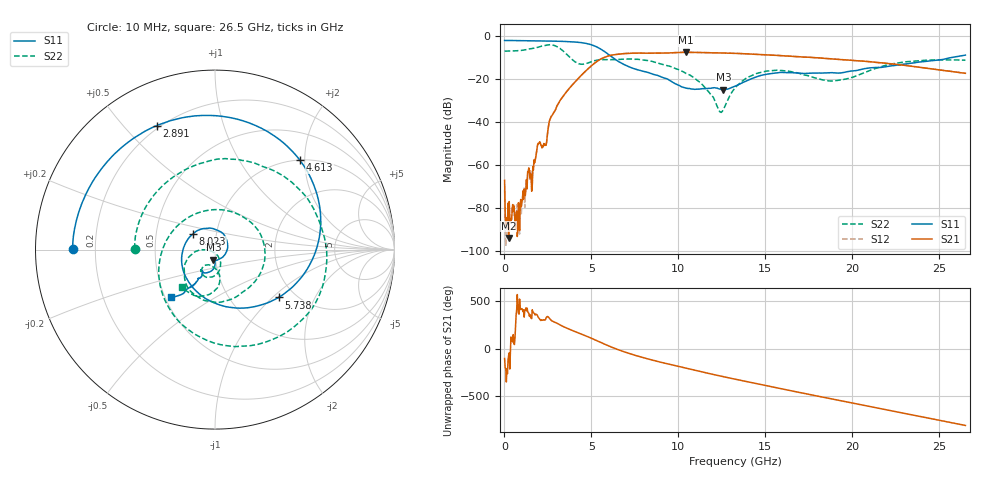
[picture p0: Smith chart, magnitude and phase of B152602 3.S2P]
!  2-Port S-parameters saved by WinCal
! VAR MeasName=S-Parameters (CALIBRATED_DATA) read from VNA (N5242A)
! VAR MeasDate=2016-1-5 16:25:45
! VAR NAME=B152602 3
! VAR FILENAME=B152602 3.S2P
! VAR DATE=2016-1-5 16:25:45
! VAR PHYS_PORTS=1,2
# Hz S DB R 50
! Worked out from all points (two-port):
!   801 points, 10 MHz to 26.5 GHz, reference 50 ohm
!   highest |S21| = -7.52 dB at 10.44 GHz (marker M1); lowest = -93.8 dB at 241.8 MHz (marker M2)
!   |S21| within 3 dB of the highest: 5.573 GHz to 18.72 GHz (13.14 GHz wide, 108 % of centre)
!   lowest |S11| = -24.9 dB at 12.59 GHz (marker M3), VSWR 1.12, Z = 48.8 - j5.54 ohm
!   |S11| at or under -10 dB: 6.233 GHz to 25.66 GHz (19.43 GHz wide, 122 % of centre)
!   |S22| runs from -35.5 to -4.0 dB; largest |S21 - S12| = 0.0029
!   S11 on the Smith chart (normalised r, x): 10 MHz: 0.12, +0.00; 2.891 GHz: 0.19, +0.62; 4.613 GHz: 1.00, +1.89; 5.738 GHz: 1.65, -1.09; 8.023 GHz: 0.77, +0.14; 26.5 GHz: 0.54, -0.33
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1e7  -2.01 179.7  -67.03 -100.5  -71.39 93.6  -6.98 179.4
2.417875e8  -2.02 175.0  -93.79 -67.0  -93.05 152.2  -6.95 165.2
8.70925e8  -2.10 162.1  -90.33 164.8  -91.99 -123.5  -6.71 126.0
1.764962e9  -2.20 143.2  -57.81 -2.8  -57.58 -0.4  -5.49 62.8
2.460325e9  -2.29 126.8  -46.48 -18.4  -46.42 -18.6  -4.12 -0.8
2.890788e9  -2.34 115.2  -34.82 -79.5  -34.80 -79.4  -4.40 -53.1
3.58615e9  -2.51 93.1  -25.70 -140.8  -25.73 -140.8  -8.49 -142.5
4.447075e9  -3.05 55.6  -18.00 154.4  -18.01 154.5  -13.07 97.5
4.612638e9  -3.26 46.5  -16.65 142.4  -16.67 142.5  -12.89 75.8
5.17555e9  -4.54 9.2  -12.60 98.8  -12.59 98.9  -11.39 15.2
5.738462e9  -7.06 -37.0  -9.90 52.4  -9.88 52.5  -10.90 -26.7
6.731838e9  -12.61 -127.8  -8.20 -20.4  -8.20 -20.4  -10.75 -69.3
8.023225e9  -16.41 143.9  -7.92 -94.2  -7.92 -94.2  -11.14 -112.3
8.851038e9  -18.40 98.8  -7.87 -133.4  -7.88 -133.6  -12.59 -136.0
1.044044e10  -24.13 -26.0  -7.52 156.6  -7.52 156.8  -17.34 -167.6
1.259275e10  -24.85 -98.5  -7.85 68.1  -7.84 67.9  -34.00 -94.9
1.3255e10  -23.27 -90.7  -8.01 42.0  -8.01 41.9  -24.06 -65.2
1.504308e10  -17.77 -104.4  -8.71 -26.8  -8.71 -27.0  -16.29 -96.0
1.769208e10  -17.19 -123.6  -9.91 -125.0  -9.88 -124.9  -19.00 -124.1
1.957949e10  -16.73 -118.2  -11.04 166.6  -11.02 166.6  -20.04 -92.8
2.209604e10  -14.00 -119.4  -12.77 74.8  -12.71 74.6  -13.23 -87.7
2.65e10  -8.82 -132.7  -17.27 -85.1  -17.26 -85.4  -11.19 -131.7
